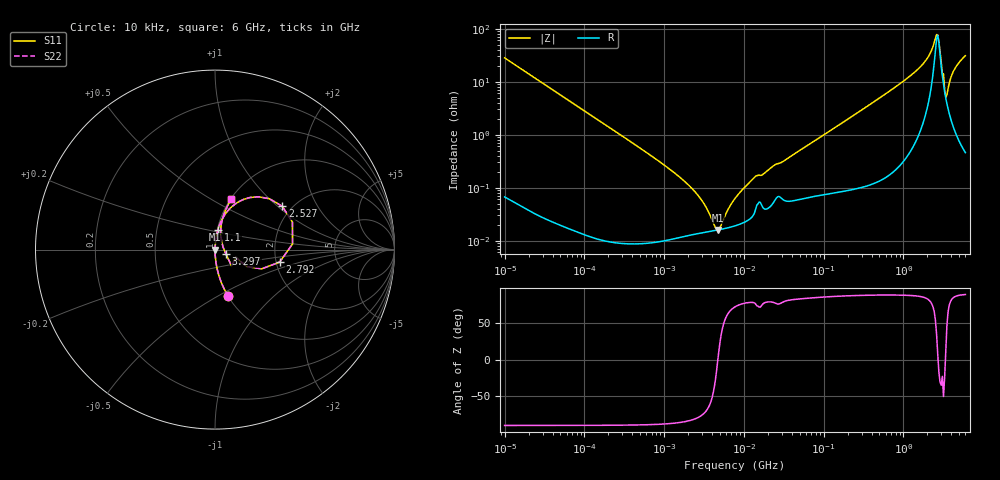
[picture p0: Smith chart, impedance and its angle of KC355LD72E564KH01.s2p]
!Murata Part Number: KC355LD72E564KH01
!These Parameters are Measured in Series Mode Connection
!Data Generated on Jun 19, 2026
!  o--ll--o
!Port1  Port2
!  o------o
!Operation Temp=25[degC], DC Bias Voltage=0[V]
!Freq. Start=10[kHz] Stop=6[GHz] 401[Steps]
# Hz S RI R 50
!Freq.(Hz) S11(Real) S11(Imag) S21(Real) S21(Imag) S12(Real) S12(Imag) S22(Real) S22(Imag)
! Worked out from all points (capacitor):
!   401 points, 10 kHz to 6 GHz, reference 50 ohm
!   read as one part in series: C = 566 nF near 10.69 kHz
!   lowest |Z| = 15.9 mohm at 4.703 MHz (marker M1)
!   series resonance near 4.72 MHz, so ESL is about 2 nH
!   S11 on the Smith chart (normalised r, x): 10 kHz: 1.00, -0.56; 1.1 GHz: 1.01, +0.23; 2.527 GHz: 1.78, +1.07; 2.792 GHz: 2.09, -0.34; 3.297 GHz: 1.13, -0.06; 6 GHz: 1.01, +0.62
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10000  0.0738 -0.2603  0.9262 0.2603  0.9262 0.2603  0.0738 -0.2603
27124  0.011 -0.1027  0.989 0.1027  0.989 0.1027  0.011 -0.1027
92862  0.00106 -0.0303  0.9989 0.0303  0.9989 0.0303  0.00106 -0.0303
862344  0.000105 -0.00314  0.9999 0.00314  0.9999 0.00314  0.000105 -0.00314
2499958  0.000134 -0.000791  0.9999 0.000791  0.9999 0.000791  0.000134 -0.000791
3155371  0.000142 -0.00048  0.9999 0.00048  0.9999 0.00048  0.000142 -0.00048
4256561  0.000154 -0.00012  0.9998 0.00012  0.9998 0.00012  0.000154 -0.00012
4703216  0.000159 -4.1e-06  0.9998 4.1e-06  0.9998 4.1e-06  0.000159 -4.1e-06
7745967  0.00019 0.000595  0.9998 -0.000595  0.9998 -0.000595  0.00019 0.000595
1.409589e7  0.000401 0.0016  0.9996 -0.0016  0.9996 -0.0016  0.000401 0.0016
7.193098e7  0.000721 0.0071  0.9993 -0.0071  0.9993 -0.0071  0.000721 0.0071
6.67969e8  0.00603 0.0654  0.994 -0.0654  0.994 -0.0654  0.00603 0.0654
1.100112e9  0.0164 0.1114  0.9836 -0.1114  0.9836 -0.1114  0.0164 0.1114
1.936459e9  0.0832 0.229  0.9168 -0.229  0.9168 -0.229  0.0832 0.229
2.286837e9  0.1955 0.2903  0.8045 -0.2903  0.8045 -0.2903  0.1955 0.2903
2.526803e9  0.3746 0.2414  0.6254 -0.2414  0.6254 -0.2414  0.3746 0.2414
2.791949e9  0.3604 -0.0695  0.6396 0.0695  0.6396 0.0695  0.3604 -0.0695
2.983997e9  0.1747 -0.0939  0.8253 0.0939  0.8253 0.0939  0.1747 -0.0939
3.297118e9  0.061 -0.0246  0.939 0.0246  0.939 0.0246  0.061 -0.0246
3.523913e9  0.0381 0.0393  0.9619 -0.0393  0.9619 -0.0393  0.0381 0.0393
4.447775e9  0.041 0.1688  0.959 -0.1688  0.959 -0.1688  0.041 0.1688
6e9  0.0906 0.2798  0.9094 -0.2798  0.9094 -0.2798  0.0906 0.2798
